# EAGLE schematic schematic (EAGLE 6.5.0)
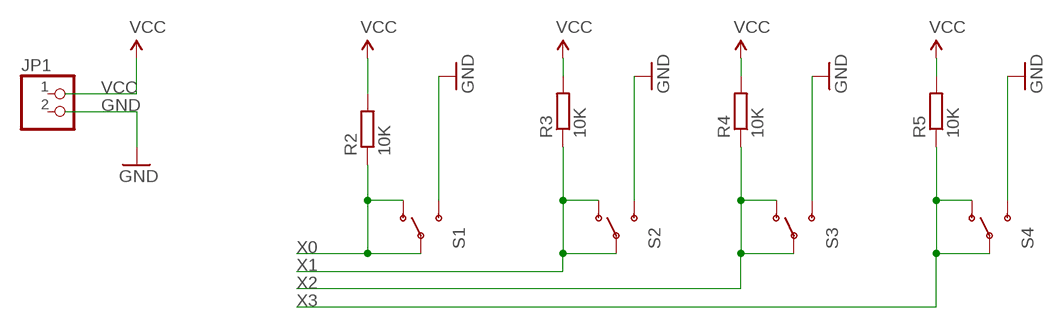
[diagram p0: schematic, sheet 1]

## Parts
JP1  PINHD-1X2  [1X02]
R2  10K  R-EU_R0805  [R0805]
R3  10K  R-EU_R0805  [R0805]
R4  10K  R-EU_R0805  [R0805]
R5  10K  R-EU_R0805  [R0805]
S1  SWITCH-SPDTPTH  [SWITCH-SPDT]
S2  SWITCH-SPDTPTH  [SWITCH-SPDT]
S3  SWITCH-SPDTPTH  [SWITCH-SPDT]
S4  SWITCH-SPDTPTH  [SWITCH-SPDT]

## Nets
GND: S1.3(S) S2.3(S) S3.3(S) S4.3(S)
VCC: R2.2 R3.2 R4.2 R5.2
X0: R2.1 S1.1(O) S1.2(P)
X1: R3.1 S2.1(O) S2.2(P)
X2: R4.1 S3.1(O) S3.2(P)
X3: R5.1 S4.1(O) S4.2(P)
Unconnected: JP1.1 JP1.2

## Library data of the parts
JP1 = pinhead:PINHD-1X2: PIN HEADER
R2-R5 = resistor:R-EU_: RESISTOR, European symbol
S1-S4 = SparkFun-Electromechanical:SWITCH-SPDT: SPDT Switch Simple slide switch, Spark Fun Electronics SKU : COM-00102 DPDT SMT slide switch, AYZ0202, SWCH-08179; PROD_ID: SWCH-08261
